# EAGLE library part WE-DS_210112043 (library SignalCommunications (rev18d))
WE-DS D-SUB-Filter Connectors Bent 90° Characteristics Standard type filtered with 1000 pF High attenuation of more than 40 dB @ 180 MHz Choice of earthing metal sheet or high speed earthing clip Rated voltage: 100 VDC Rated current @ 20 ºC: 5 A Withstand voltage: 250 VRMS Insulation resistance: min. 1000 MΩ Operating temperature: –55 ºC to +125 ºC Applications Filtering of interfaces External connection to -printer -sensor -display Details see: http://katalog.we-online.de/en/pbs/Filter_abgewinkelt Created on 2015-05-04 2015 (C) Wurth Elektronik
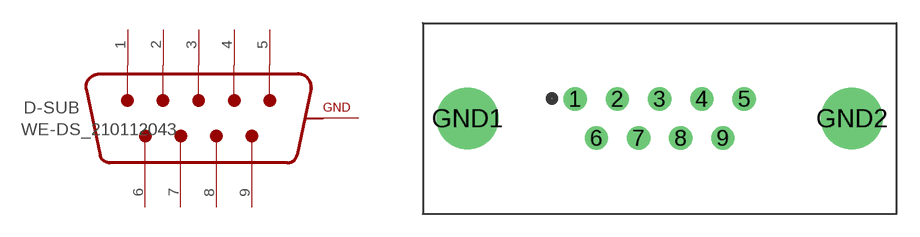
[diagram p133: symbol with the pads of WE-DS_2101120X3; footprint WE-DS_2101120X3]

Designator prefix D-SUB

## WE-DS_210112043 (WE-NUMBER: 210112043/9pins_male)  [WE-DS_2101120X3]
1  1  pas
2  2  pas
3  3  pas
4  4  pas
5  5  pas
6  6  pas
7  7  pas
8  8  pas
9  9  pas
GND1  GND  pwr
GND2  GND  pwr

## Footprint WE-DS_2101120X3 (pad centres in mm)
drill 1: 1 -5.49,1.27; 2 -2.74,1.27; 3 0,1.27; 4 2.74,1.27; 5 5.49,1.27; 6 -4.11,-1.27; 7 -1.37,-1.27; 8 1.37,-1.27; 9 4.11,-1.27
drill 3: GND1 -12.5,0; GND2 12.5,0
